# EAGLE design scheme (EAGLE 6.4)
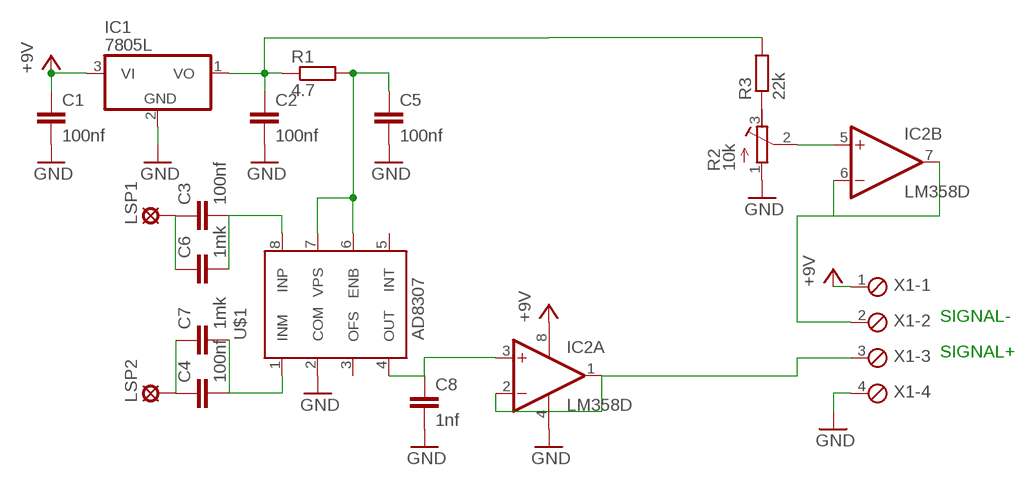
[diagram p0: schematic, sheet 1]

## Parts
C1  100nf  C-EUC0805K  [C0805K]
C2  100nf  C-EUC0805K  [C0805K]
C3  100nf  C-EUC0805K  [C0805K]
C4  100nf  C-EUC0805K  [C0805K]
C5  100nf  C-EUC0805K  [C0805K]
C6  1mk  C-EUC0805K  [C0805K]
C7  1mk  C-EUC0805K  [C0805K]
C8  1nf  C-EUC0805K  [C0805K]
IC1  7805L  [TO92]
IC2  LM358D  [SO08]
LSP1  SE14  [SE14]
LSP2  SE14  [SE14]
R1  4.7  R-EU_M0805  [M0805]
R2  10k  R-TRIMM64W  [RTRIM64W]
R3  22k  R-EU_M0805  [M0805]
U$1  AD8307  [SO8]
X1  MPT4  [4POL254]

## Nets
GND: C1.2 C2.2 C5.2 C8.2 IC1.2(GND) IC2.4(P:V-) R2.1(E) U$1.2(COM) X1.4
N$1: C2.1 IC1.1(VO) R1.1 R3.2
N$2: IC2.6(B:-IN) IC2.7(B:OUT) X1.2
N$3: C5.1 R1.2 U$1.6(ENB) U$1.7(VPS)
N$4: C3.2 C6.2 U$1.8(INP)
N$5: C4.2 C7.2 U$1.1(INM)
N$6: C4.1 C7.1 LSP2.MP
N$7: C3.1 C6.1 LSP1.MP
N$8: IC2.1(A:OUT) IC2.2(A:-IN) X1.3
N$10: C8.1 IC2.3(A:+IN) U$1.4(OUT)
N$11: IC2.5(B:+IN) R2.2(S)
N$12: R2.3(A) R3.1
VCC: C1.1 IC1.3(VI) IC2.8(P:V+) X1.1 ; supply symbol labelled +9V
Unconnected: U$1.3(OFS) U$1.5(INT)

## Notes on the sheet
- SIGNAL-
- SIGNAL+

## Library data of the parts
C1-C8 = rcl:C-EU: CAPACITOR, European symbol
IC1 = linear:78*: Positive VOLTAGE REGULATOR Source: http://cache.national.com/ds/LM/LM78L05.pdf http://www.fairchildsemi.com/ds/LM/LM7805.pdf
IC2 = linear:LM358: OP AMP also LM158; LM258; LM2904 Source: http://cache.national.com/ds/LM/LM158.pdf
LSP1 LSP2 = solpad:SE14: SOLDER PAD
R1 R3 = rcl:R-EU_: RESISTOR, European symbol
R2 = resistor:R-TRIMM: Trimm resistor
U$1 = balmer:AD8307
X1 = con-phoenix-254:MPT4: PHOENIX CONNECTOR; OC_FARNELL: unknown; OC_NEWARK: unknown

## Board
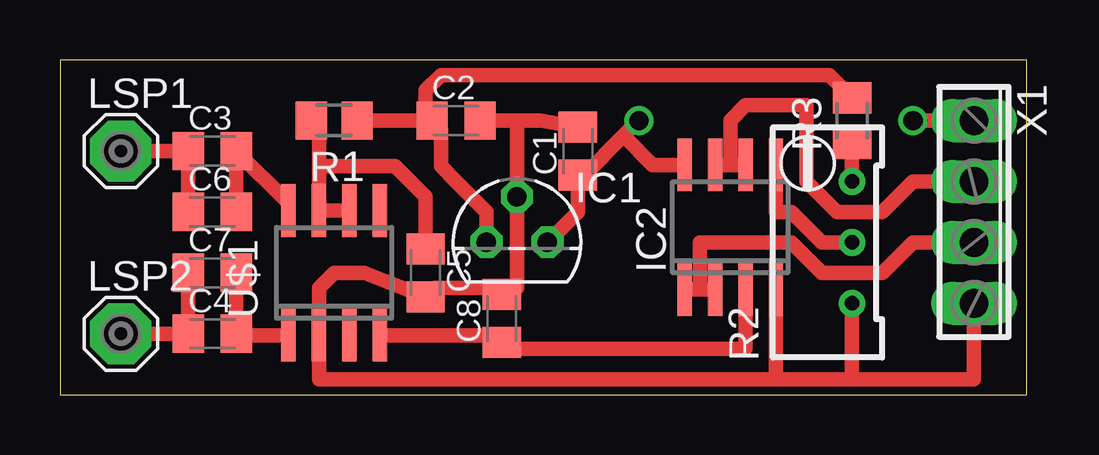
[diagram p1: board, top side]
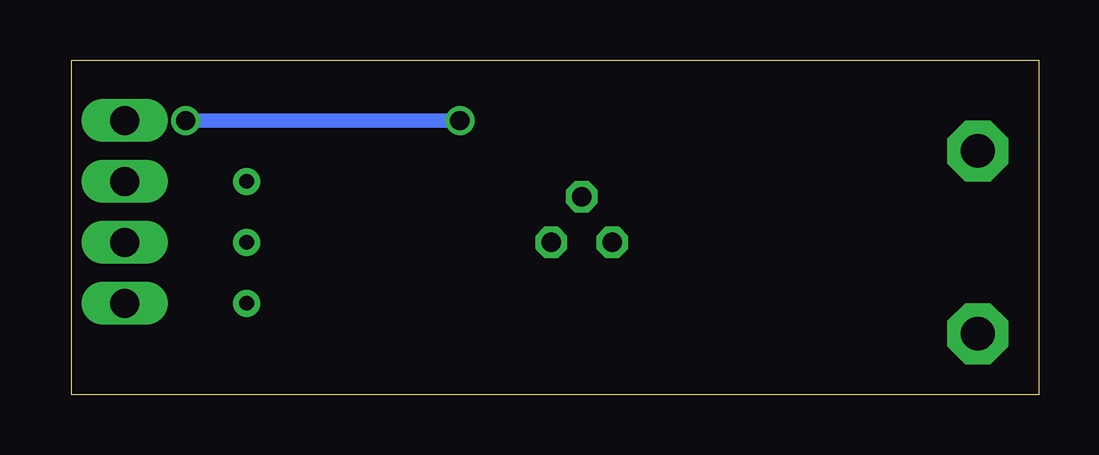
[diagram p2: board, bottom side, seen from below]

Size 40.31 x 13.96 mm. Coordinates in mm from the lower left corner, seen from the top.
Outline: 0,0 40.31,0 40.31,13.96 0,13.96 0,0
Copper layers (1*16): Top 0.035mm / dielectric 1.5mm / Bottom 0.035mm
Design rules "default": minimum track width 10mil, minimum drill 24mil, track to track 8mil, track to pad 8mil, pad to pad 8mil, via to via 8mil, smd to smd 8mil, copper to edge 40mil, drill to drill 8mil, minimum pad ring 10mil, minimum via ring 8mil, stop-mask expansion 4mil, vias tented up to drill 0mil, thermal gap 10mil

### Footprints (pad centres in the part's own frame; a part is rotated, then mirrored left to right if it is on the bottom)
C0805K = smd 1.3 x 1.6: 1 -1,0; 2 1,0
TO92 = drill 0.813 octagon: 1 -1.27,0; 2 0,1.905; 3 1.27,0
SO08 = smd 0.6 x 2.2: 1 -1.905,-2.6; 2 -0.635,-2.6; 3 0.635,-2.6; 4 1.905,-2.6; 5 1.905,2.6; 6 0.635,2.6; 7 -0.635,2.6; 8 -1.905,2.6
SE14 = drill 1.397 pad 2.54 octagon: MP 0,0
M0805 = smd 1.3 x 1.6: 1 -0.95,0; 2 0.95,0
RTRIM64W = drill 0.61: 1 1.27,-2.54; 2 1.27,0; 3 1.27,2.54
SO8 = smd 0.6 x 2.2: 1 -1.905,-2.6; 2 -0.635,-2.6; 3 0.635,-2.6; 4 1.905,-2.6; 5 1.905,2.6; 6 0.635,2.6; 7 -0.635,2.6; 8 -1.905,2.6
4POL254 = drill 1.2 long: 1 -3.81,0; 2 -1.27,0; 3 1.27,0; 4 3.81,0

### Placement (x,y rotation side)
C1  21.59,10.16 90 top
C2  16.51,11.43 0 top
C3  6.35,10.16 0 top
C4  6.35,2.54 0 top
C5  15.24,5.08 270 top
C6  6.35,7.62 0 top
C7  6.35,5.08 0 top
C8  18.41,3.17 90 top
IC1  19.05,6.35 0 top
IC2  27.94,6.99 0 top
LSP1  2.54,10.16 0 top
LSP2  2.54,2.54 0 top
R1  11.43,11.43 180 top
R2  31.75,6.35 0 top
R3  33.02,11.43 90 top
U$1  11.43,5.08 0 top
X1  38.1,7.62 270 top

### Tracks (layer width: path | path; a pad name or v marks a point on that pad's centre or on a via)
GND
  Top 0.61: C2.2 19.05,11.43 | 19.05,11.43 20.05,11.43 C1.2 | C5.2 14.97,4.08 | 19.05,4.45 IC1.2 19.05,11.43 | 19.05,4.45 15.61,4.45 C5.2 | 29.84,0.64 10.79,0.64 U$1.2 10.79,4.45 11.43,5.08 12.7,5.08 C5.2 | 29.84,0.64 33.02,0.64 | 33.02,0.64 38.1,0.64 X1.4 | 19.05,4.45 18.68,4.45 C8.2 | IC2.4 29.84,0.64 | R2.1 33.02,0.64
N$1
  Top 0.61: 15.24,11.43 R1.1 15.24,11.43 | 15.24,11.43 C2.1 15.88,11.06 15.88,9.53 16.51,8.89 17.78,7.62 IC1.1 | 15.24,11.43 15.24,12.7 15.88,13.34 26.04,13.34 32.06,13.34 R3.2
N$2
  Top 0.61: IC2.7 27.94,9.59 | 27.94,9.59 IC2.6 | X1.2 35.56,8.89 34.29,7.62 32.38,7.62 31.11,8.89 31.11,12.06 28.57,12.06 27.94,11.43 27.94,9.59
N$3
  Top 0.61: U$1.6 U$1.7 10.79,9.53 | 10.79,9.53 10.79,10.16 10.79,11.12 R1.2 | C5.1 15.24,8.26 13.97,9.53 10.79,9.53
N$4
  Top 0.61: U$1.8 9.53,7.99 C3.2 C6.2
N$5
  Top 0.61: U$1.1 7.41,2.48 C4.2 C7.2
N$6
  Top 0.61: LSP2.MP C4.1 C7.1
N$7
  Top 0.61: LSP1.MP C3.1 C6.1
N$8
  Top 0.61: IC2.1 26.67,4.38 | 26.67,4.38 IC2.2 | X1.3 35.56,6.35 34.29,5.08 31.75,5.08 30.48,6.35 26.67,6.35 26.67,4.38
N$10
  Top 0.61: U$1.4 18.11,2.48 C8.1 18.68,1.91 28.57,1.91 IC2.3
N$11
  Top 0.61: R2.2 31.75,6.35 30.48,7.62 29.84,7.62 IC2.5
N$12
  Top 0.61: R2.3 R3.1
VCC  (via drill 0.8)
  Top 0.61: IC1.3 21.59,7.62 C1.1 21.86,9.16 23.5,10.79 | 23.5,10.79 v24.13,11.43 | v35.56,11.43 X1.1 | IC2.8 24.7,9.59 23.5,10.79
  Bottom 0.61: v24.13,11.43 v35.56,11.43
